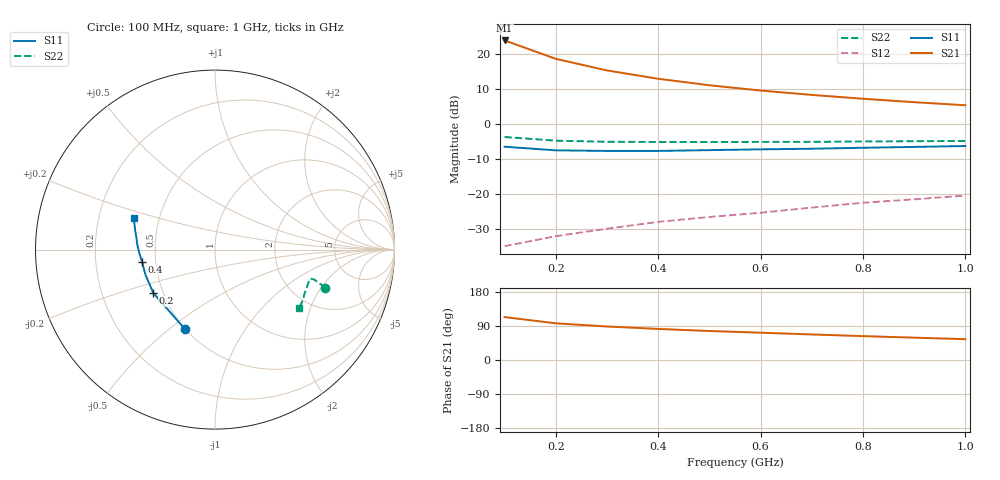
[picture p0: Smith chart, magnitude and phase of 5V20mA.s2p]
#  HZ  S  MA  R  50.0000
! Device:15GN03CA
! "! Bias:VCE=5V, IC=20mA  "
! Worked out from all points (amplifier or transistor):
!   10 points, 100 MHz to 1 GHz, reference 50 ohm
!   highest |S21| = 23.8 dB at 100 MHz (marker M1)
!   |S21| within 3 dB of that: start of sweep to 157.2 MHz
!   unconditionally stable (mu >= 1): 147.8 MHz to end of sweep
!   at 200 MHz: K = 1.23, MAG = 22.4 dB, |S12| = -32.0 dB
!   at 600 MHz: K = 1.58, MAG = 13.0 dB, |S12| = -25.4 dB
!   at 1 GHz: K = 1.29, MAG = 9.7 dB, |S12| = -20.4 dB
!   S11 on the Smith chart (normalised r, x): 100 MHz: 0.50, -0.57; 200 MHz: 0.44, -0.26; 400 MHz: 0.42, -0.07; 1 GHz: 0.36, +0.16
1e8  0.473 -110.9  15.55 113.2  0.018 48.8  0.651 -19.0
2e8  0.42 -145.0  8.504 96.8  0.025 55.5  0.577 -16.8
3e8  0.412 -160.5  5.806 88.4  0.032 64.3  0.556 -16.9
4e8  0.412 -170.5  4.415 82.0  0.04 69.4  0.553 -18.4
5e8  0.423 -177.8  3.567 76.5  0.047 73.5  0.552 -20.6
6e8  0.434 176.3  2.998 72.1  0.054 76.9  0.554 -23.2
7e8  0.443 171.3  2.597 67.4  0.064 79.4  0.555 -25.8
8e8  0.457 166.6  2.289 63.0  0.075 80.2  0.562 -28.8
9e8  0.47 162.6  2.044 59.0  0.084 82.6  0.567 -31.9
1e9  0.484 159.0  1.849 55.0  0.095 83.6  0.572 -34.9
